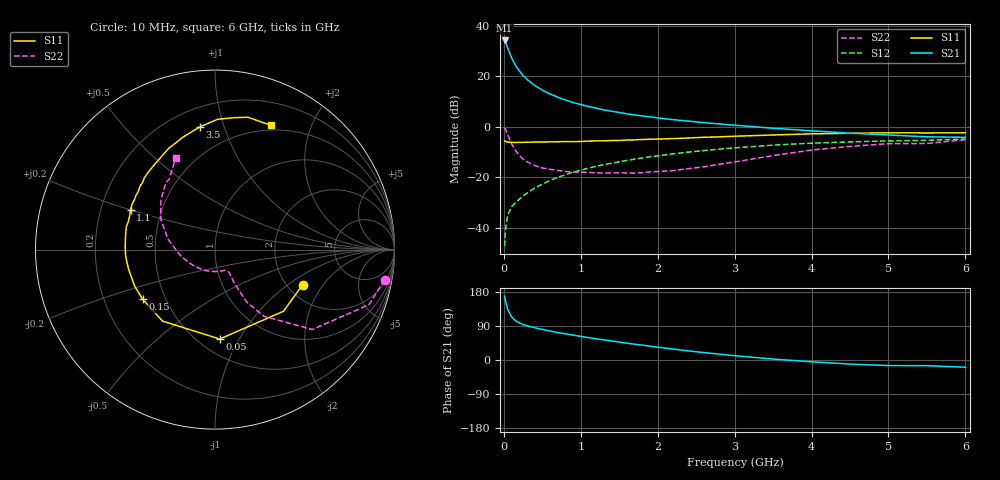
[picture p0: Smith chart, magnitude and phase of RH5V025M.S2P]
! SIEMENS Small Signal Semiconductors
! BFR106
! Si NPN RF Bipolar Junction Transistor in SOT23
! VCE = 5 V  IC = 25 mA
! Common Emitter S-Parameters:  August  1996
# GHz  S  MA  R  50
!  f  S11  S21  S12  S22
! GHz  MAG  ANG  MAG  ANG  MAG  ANG  MAG  ANG
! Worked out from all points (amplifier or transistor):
!   36 points, 10 MHz to 6 GHz, reference 50 ohm
!   highest |S21| = 34.2 dB at 10 MHz (marker M1)
!   |S21| within 3 dB of that: start of sweep to 50.68 MHz
!   unconditionally stable (mu >= 1): 348.4 MHz to 2.146 GHz
!   at 250 MHz: K = 0.93, MSG = 23.9 dB, |S12| = -27.5 dB
!   at 1.4 GHz: K = 1.06, MAG = 8.8 dB, |S12| = -14.4 dB
!   at 6 GHz: K = 0.99, MSG = 0.3 dB, |S12| = -4.8 dB
!   S11 on the Smith chart (normalised r, x): 10 MHz: 2.41, -1.31; 50 MHz: 0.63, -0.83; 150 MHz: 0.37, -0.27; 1.1 GHz: 0.33, +0.20; 3.5 GHz: 0.32, +0.83; 6 GHz: 0.44, +1.46
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0.01  0.5261 -21.9  51.56 167.4  0.0043 82.4  0.9601 -10.1
0.02  0.5134 -42.0  48.57 157.2  0.0089 74.5  0.9107 -19.7
0.05  0.4989 -87.0  36.73 133.6  0.0176 60.9  0.7016 -39.4
0.1  0.4942 -126.3  23.58 114.2  0.0259 55.9  0.4612 -53.7
0.15  0.4885 -145.6  16.69 103.8  0.0313 56.0  0.3392 -58.9
0.2  0.4919 -155.4  12.91 98.2  0.0366 59.2  0.2736 -59.4
0.25  0.4907 -162.7  10.41 93.5  0.0424 61.2  0.2287 -59.7
0.3  0.4942 -168.1  8.747 90.4  0.0483 63.7  0.2044 -59.9
0.4  0.4993 -175.8  6.639 85.2  0.061 66.1  0.1708 -58.9
0.5  0.5003 178.5  5.34 80.6  0.073 67.3  0.1526 -58.2
0.6  0.5027 173.2  4.486 76.5  0.0863 67.7  0.1439 -59.2
0.7  0.5061 169.1  3.874 72.5  0.0991 68.1  0.1367 -61.2
0.9  0.5074 161.9  3.041 65.6  0.1259 66.9  0.1267 -64.8
1.1  0.5206 154.7  2.536 59.1  0.1514 65.5  0.1245 -72.6
1.3  0.5278 148.4  2.169 53.1  0.1778 63.4  0.1211 -80.3
1.6  0.5464 139.9  1.809 44.4  0.2158 60.0  0.1217 -95.2
2.2  0.5844 124.5  1.387 28.9  0.2912 52.1  0.1358 -129.1
2.8  0.6322 110.5  1.142 15.5  0.3607 43.3  0.181 -164.1
3.5  0.6885 97.2  0.936 2.5  0.4336 32.8  0.2692 167.3
4.5  0.7425 81.8  0.749 -10.7  0.5025 17.4  0.4092 137.5
5.5  0.7564 69.7  0.634 -15.0  0.5393 7.1  0.4671 123.1
6  0.7607 65.6  0.62 -19.0  0.5737 -0.4  0.5574 113.1
